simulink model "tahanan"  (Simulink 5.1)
settings: Solver=ode45  StartTime=0.0  StopTime=10  RelTol=1e-3

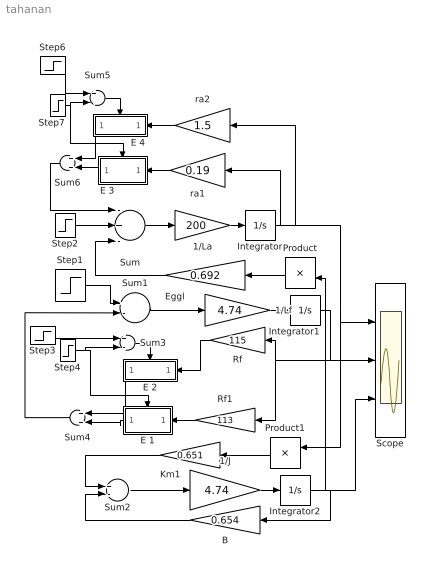
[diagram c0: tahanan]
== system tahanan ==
  1/J : Gain  Gain=4.74
  1/La : Gain  Gain=200
  1/Lf : Gain  Gain=4.74
  B : Gain  Orientation=left  Gain=0.654
  E 1 : Subsystem  Orientation=left  TreatAsAtomicUnit=on
  E 2 : Subsystem  Orientation=left  TreatAsAtomicUnit=on
  E 3 : Subsystem  Orientation=left  TreatAsAtomicUnit=on
  E 4 : Subsystem  Orientation=left  TreatAsAtomicUnit=on
  Eggl : Gain  Orientation=left  Gain=0.692
  Integrator : Integrator
  Integrator1 : Integrator
  Integrator2 : Integrator
  Km1 : Gain  Orientation=left  Gain=0.651
  Product : Product  Orientation=left
  Product1 : Product  Orientation=left
  Rf : Gain  Orientation=left  Gain=115
  Rf1 : Gain  Orientation=left  Gain=113
  Scope : Scope  NumInputPorts=3
  Step1 : Step  Time=0  After=300  SampleTime=0
  Step2 : Step  Time=0  After=500  SampleTime=0
  Step3 : Step  Time=0  SampleTime=0
  Step4 : Step  SampleTime=0
  Step6 : Step  Time=0  SampleTime=0
  Step7 : Step  SampleTime=0
  Sum : Sum  Inputs=-+-
  Sum{1..3,5} (4 alike) : Sum  Inputs=+-
  Sum4 : Sum  Orientation=left
  Sum6 : Sum  Orientation=left
  ra1 : Gain  Orientation=left  Gain=0.19
  ra2 : Gain  Orientation=left  Gain=1.5
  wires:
  Sum/1 -> 1/La/1
  1/La/1 -> Integrator/1
  Integrator/1 -> ra2/1, Product1/1, Scope/1, ra1/1
  Product/1 -> Eggl/1
  Sum1/1 -> 1/Lf/1
  1/Lf/1 -> Integrator1/1
  Integrator1/1 -> Rf/1, Rf1/1, Scope/2
  1/J/1 -> Integrator2/1
  Product1/1 -> Km1/1
  Km1/1 -> Sum2/1
  B/1 -> Sum2/2
  Step1/1 -> Sum1/1
  Step4/1 -> Sum3/2, E 1/Enable
  Step3/1 -> Sum3/1
  Rf1/1 -> E 1/1(In1)
  E 1/1(Out1) -> Sum4/2
  Sum3/1 -> E 2/Enable
  Rf/1 -> E 2/1(In1)
  E 2/1(Out1) -> Sum4/1
  Sum4/1 -> Sum1/2
  Step7/1 -> Sum5/2, E 3/Enable
  Step6/1 -> Sum5/1
  E 3/1(Out1) -> Sum6/2
  Sum5/1 -> E 4/Enable
  E 4/1(Out1) -> Sum6/1
  ra1/1 -> E 3/1(In1)
  ra2/1 -> E 4/1(In1)
  Sum6/1 -> Sum/1
  Step2/1 -> Sum/2
  Eggl/1 -> Sum/3
  Integrator2/1 -> Scope/3, B/1, Product/2
  Sum2/1 -> 1/J/1

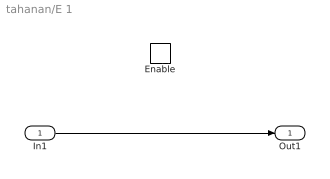
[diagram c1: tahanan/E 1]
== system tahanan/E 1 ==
  In1 : Inport
  Enable : EnablePort
  Out1 : Outport  OutputWhenDisabled=reset  InitialOutput=[0]
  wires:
  In1/1 -> Out1/1

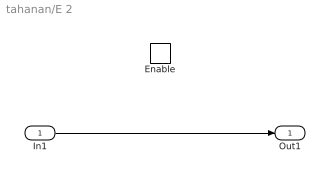
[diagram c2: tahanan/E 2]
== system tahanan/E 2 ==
  In1 : Inport
  Enable : EnablePort
  Out1 : Outport  OutputWhenDisabled=reset  InitialOutput=[0]
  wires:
  In1/1 -> Out1/1

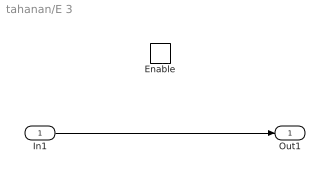
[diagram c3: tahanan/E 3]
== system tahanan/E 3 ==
  In1 : Inport
  Enable : EnablePort
  Out1 : Outport  OutputWhenDisabled=reset  InitialOutput=[0]
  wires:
  In1/1 -> Out1/1

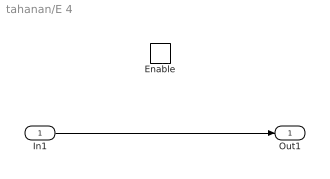
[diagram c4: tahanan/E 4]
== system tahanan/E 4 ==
  In1 : Inport
  Enable : EnablePort
  Out1 : Outport  OutputWhenDisabled=reset  InitialOutput=[0]
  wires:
  In1/1 -> Out1/1
